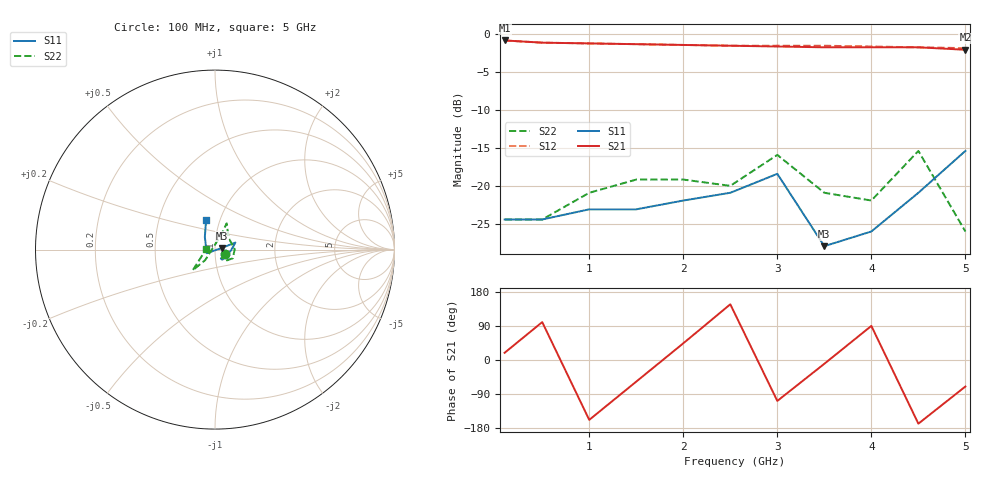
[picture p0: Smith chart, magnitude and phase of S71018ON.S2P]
!  MGS-71018 S PARAMETERS
!  "on" port  LAST UPDATED 07-22-92
# ghz s ma r 50
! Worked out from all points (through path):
!   11 points, 100 MHz to 5 GHz, reference 50 ohm
!   highest |S21| = -0.82 dB at 100 MHz (marker M1); lowest = -2.0 dB at 5 GHz (marker M2)
!   lowest |S11| = -28.0 dB at 3.5 GHz (marker M3), VSWR 1.08, Z = 54 + j1.05 ohm
!   |S11| at or under -10 dB: start of sweep to end of sweep
!   |S22| runs from -26.0 to -15.4 dB; largest |S21 - S12| = 0.029
0.1  0.06 -22.0  0.91 19.0  0.91 19.0  0.06 -24.0
0.5  0.06 -57.0  0.88 100.0  0.88 100.0  0.06 -52.0
1  0.07 -54.0  0.87 -158.0  0.87 -159.0  0.09 -42.0
1.5  0.07 -17.0  0.86 -57.0  0.86 -57.0  0.11 -26.0
2  0.08 -14.0  0.85 44.0  0.85 44.0  0.11 1.0
2.5  0.09 -2.0  0.84 147.0  0.84 147.0  0.1 41.0
3  0.12 19.0  0.83 -108.0  0.84 -108.0  0.16 66.0
3.5  0.04 14.0  0.82 -10.0  0.84 -9.0  0.09 67.0
4  0.05 -156.0  0.82 90.0  0.83 90.0  0.08 -133.0
4.5  0.09 129.0  0.82 -168.0  0.82 -170.0  0.17 -137.0
5  0.17 107.0  0.79 -70.0  0.81 -71.0  0.05 178.0
